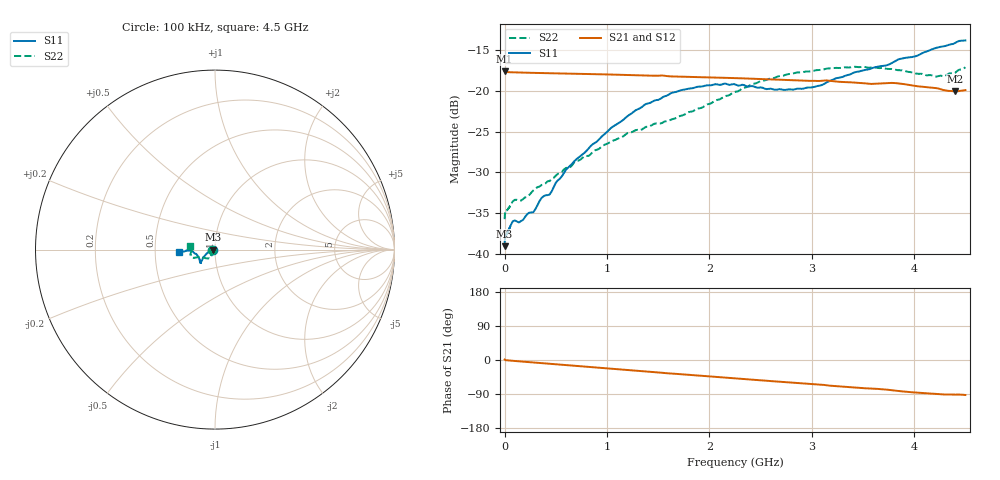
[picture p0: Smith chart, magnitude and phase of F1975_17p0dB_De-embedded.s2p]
! Integrated Device Technology
! Corporate Headquarters
! 6024 Silver Creek Valley Road
! San Jose, CA 95138  USA
! Phone:  1-408-284-8200
! Toll Free:  1-800-223-1366
! Webpage:  http://www.idt.com/
! Timing and RF Division
! 515 Groton Road, Suite 102
! Westford, MA 01886-6024
! Device:  F1975
! Description: 6-bit, 75 ohm, 0.5 dB Digital Step Attenuator
! Frequency:  5.0 MHz -  3.00 GHz
! Package:  4x4 mm QFN Plastic Package: 20 pin
! Ports:  2 RF, 11 DC
!  Pin  1  = D5 (16 dB)
!  Pin  2  = RF1  =  Port 1
!  Pin  3  = Serial Data In (DATA)
!  Pin  4  = Serial Clock (CLK)
!  Pin  5  = Serial Latch Enable (LE)
!  Pin  6  = VDD
!  Pin  7  = NC
!  Pin  8  = NC
!  Pin  9  = NC
!  Pin 10  = GND
!  Pin 11  = GND
!  Pin 12  = NC
!  Pin 13  = VMODE
!  Pin 14  = RF2  =  Port 2
!  Pin 15  = D4 (8 dB)
!  Pin 16  = D3 (4 dB)
!  Pin 17  = D2 (2 dB)
!  Pin 18  = NC
!  Pin 19  = D1 (1 dB)
!  Pin 20  = D0 (0.5 dB)
! State:  34
! Atten State:  17.0 dB
! Voltage:  +3.30 Volts
! Current:  0.592 mA
! Data:  The device was measured on a F1975 evaluation board which has
!  individual transmission lines to the RF pins.  Data was collected
!  using a calibrated network analyzer.  The evaluation board was
!  de-embedded using Automatic Fixture Removal (AFR).
!  The reference plane is the edge of the package pin.
! Misc:
!  Action Tracker AT0415
! Date Measured:  2018-02-08
! Date:  2018-03-26  MJV
! Note:
!  Integrated Device Technology supplies this data as a sample of measured
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# GHz S dB R 75
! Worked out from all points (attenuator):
!   291 points, 100 kHz to 4.5 GHz, reference 75 ohm
!   highest |S21| = -17.65 dB at 100 kHz (marker M1); lowest = -20.1 dB at 4.4 GHz (marker M2)
!   lowest |S11| = -39.0 dB at 100 kHz (marker M3), VSWR 1.02, Z = 73.3 - j0.0127 ohm
!   |S11| at or under -10 dB: start of sweep to end of sweep
!   |S22| runs from -35.7 to -17.1 dB; largest |S21 - S12| = 0.00013
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0.0001  -39.00 -179.6  -17.65 1.2  -17.66 1.2  -35.71 -178.4
0.002  -38.18 -177.0  -17.69 0.9  -17.70 0.8  -35.24 -177.3
0.011  -37.74 -176.0  -17.72 -0.4  -17.72 -0.4  -34.82 -175.2
0.08  -35.96 -171.2  -17.77 -2.1  -17.77 -2.1  -33.52 -165.2
0.14  -36.11 -167.6  -17.79 -3.5  -17.79 -3.5  -33.42 -154.1
0.28  -34.86 -168.8  -17.83 -6.6  -17.83 -6.6  -32.20 -142.6
0.36  -33.13 -168.6  -17.86 -8.3  -17.86 -8.3  -31.53 -134.5
0.44  -32.68 -166.6  -17.88 -10.0  -17.87 -10.1  -31.05 -128.8
0.6  -29.66 -164.1  -17.92 -13.5  -17.92 -13.5  -29.45 -124.1
0.76  -27.79 -157.9  -17.96 -17.0  -17.96 -17.0  -28.22 -121.7
1.04  -24.55 -151.6  -18.04 -23.1  -18.04 -23.1  -26.23 -119.9
1.28  -22.40 -146.7  -18.12 -28.2  -18.12 -28.2  -24.83 -122.1
1.52  -21.02 -141.9  -18.16 -33.1  -18.16 -33.1  -24.03 -128.8
1.88  -19.54 -137.8  -18.35 -40.7  -18.35 -40.7  -22.21 -143.8
2.26  -19.29 -138.7  -18.48 -48.6  -18.47 -48.6  -20.13 -154.8
2.64  -19.90 -149.7  -18.65 -56.4  -18.65 -56.4  -18.43 -158.0
3.02  -19.55 -165.0  -18.81 -63.9  -18.81 -63.9  -17.57 -160.7
3.42  -17.77 -176.0  -19.02 -72.6  -19.02 -72.6  -17.09 -166.7
3.76  -16.78 -177.6  -19.06 -79.0  -19.06 -79.0  -17.37 -173.2
4.2  -14.84 -176.1  -19.68 -89.3  -19.68 -89.3  -18.29 175.3
4.4  -14.18 -174.9  -20.09 -91.4  -20.09 -91.4  -17.83 172.2
4.5  -13.88 -176.7  -19.94 -92.4  -19.94 -92.4  -17.15 170.7
